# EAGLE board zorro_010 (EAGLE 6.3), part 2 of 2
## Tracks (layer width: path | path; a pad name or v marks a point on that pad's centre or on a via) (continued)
N$8 (continued)
  Top 0.254: 32.56,16.52 33.57,16.52 33.83,16.27 33.83,15.63 33.45,15.25 | 33.45,15.25 33.83,14.87 33.83,14.23 33.57,13.98 32.56,13.98 | 33.45,15.25 33.06,15.25
N$9
  Top 0.152: R7.2 79.3,95.17 79.9,95.77 84.41,95.77 X303.B60
N$10
  Top 0.152: LED1.A R32.2
N$11
  Top 0.152: LED2.A R33.2
N$12
  Top 0.152: LED3.A R34.2
N$13
  Top 0.152: LED4.A R35.2
N$14
  Top 0.152: LED5.A R36.2
N$15
  Top 0.152: LED6.A R37.2
N$18  (via drill 0.25 pad 0.67)
  Top 0.152: R2.2 v78.1,28.17
  Bottom 0.152: v78.1,28.17 79.2,29.27 84.33,29.27 X300.A60
N$19
  Top 0.61: R300.2 26.66,63.94 VR300.5
N$20
  Top 0.152: 3.01,31.11 3.01,29.07 5.55,29.07 5.55,31.11 | 5.55,31.11 3.01,31.11 | 3.01,33.14 3.01,31.11 | 5.55,33.14 3.01,33.14 | 5.55,33.14 5.55,31.11 | 3.01,35.17 3.01,33.14 | 5.55,35.17 3.01,35.17 | 5.55,35.17 5.55,33.14 | 3.01,35.17 3.01,37.2 5.55,37.2 5.55,35.17
N$21  (via drill 0.25 pad 0.67)
  Top 0.152: R3.2 v79.8,53.57
  Bottom 0.152: X301.A60 84.37,52.27 81.1,52.27 v79.8,53.57
N$22  (via drill 0.25 pad 0.67)
  Top 0.152: R9.2 v79.8,56.07
  Bottom 0.152: X301.B60 84.34,57.37 81.1,57.37 v79.8,56.07
N$23
  POWER 0.152: 3.01,37.2 3.01,29.07 5.55,29.07 5.55,37.2 3.01,37.2
N$24
  Bottom 0.254: 35.35,16.52 34.34,16.52 34.08,16.27 34.08,15.63 34.46,15.25 | 34.46,15.25 34.08,14.87 34.08,14.23 34.34,13.98 35.35,13.98 | 34.46,15.25 34.84,15.25
N$31
  GND 0.152: 3.01,37.2 3.01,29.07 5.55,29.07 5.55,37.2 3.01,37.2
N$32A
  Bottom 0.152: 3.01,31.11 3.01,29.07 5.55,29.07 | 3.01,33.14 3.01,31.11 | 3.01,35.17 3.01,33.14 | 3.01,35.17 3.01,37.2 5.55,37.2 5.55,35.17 | 5.55,35.17 5.55,33.14 | 5.55,33.14 5.55,31.11 3.01,31.11 | 5.55,33.14 3.01,33.14 | 5.55,35.17 3.01,35.17
N$40  (via drill 0.25 pad 0.67)
  Top 0.152: R8.2 v76.8,28.17
  Bottom 0.152: X300.B60 84.35,34.37 83,34.37 v76.8,28.17
OPT0
  Top 0.152: R38.2 33.1,59.27 33.1,60.97 35.8,63.67 36.7,63.67 38,62.37 SV3.5 40.9,62.37 44.65,66.12 IC201H.10
OPT1
  Top 0.152: 34.9,59.27 36.2,60.57 SV3.3 39.8,60.57 43.35,64.12 IC201H.14 | 34.9,59.27 | R39.2 34.9,59.27
OPT2
  Top 0.152: R40.2 SV3.1 38.71,58.78 42.55,62.62 IC201H.17
P-AD0
  Top 0.152: IC200L.111 64.05,43.32 64.6,43.87 71,43.87 79.4,52.27 86.91,52.27 X301.A58
  Bottom 0.152: X303.A58 88.16,90.83 88.29,90.7 88.29,88.66 88.1,88.47 88.1,78.51 89.24,77.37 89.24,75.72 88.35,74.83 88.35,72.73 88.16,72.54 X302.A58 88.16,68.29 87.85,67.97 87.85,58.25 89.24,56.86 89.24,55.27 88.35,54.38 88.35,52.22 88.16,52.03 X301.A58 88.16,49.94 88.35,49.74 88.35,37.49 89.24,36.6 89.24,34.82 88.16,33.74 X300.A58
P-AD1
  Top 0.152: IC200L.77 70.35,24.92 74.6,29.17 74.6,30.67 80.8,36.87 86.94,36.87 X300.B58
  Bottom 0.152: X303.B58 88.16,93.81 86.89,92.54 86.89,91.27 87.97,90.19 87.97,88.85 87.7,88.57 87.7,77.96 88.16,77.49 X302.B58 88.16,75.53 87.97,75.33 87.97,73.18 86.89,72.1 86.89,70.83 85.81,69.75 85.81,68.1 86.7,67.21 86.7,57.55 X301.B58 88.16,55.08 87.97,54.89 87.97,52.79 86.89,51.71 86.89,50.38 85.62,49.11 85.62,38.19 X300.B58
P-AD2
  Top 0.152: IC200L.110 64.55,43.22 64.8,43.47 71.2,43.47 77.5,49.77 88.13,49.77 X301.A57
  Bottom 0.152: X300.A57 89.43,31.2 90.7,32.47 90.7,33.74 89.62,34.82 89.62,37.05 89.43,37.23 X301.A57 89.43,49.49 89.24,49.68 89.24,51.71 90.51,52.98 90.51,54.38 89.62,55.27 89.62,57.43 88.67,58.38 88.67,68.16 X302.A57 89.43,69.94 89.24,70.13 89.24,72.16 90.51,73.43 90.51,74.76 89.56,75.72 89.56,77.91 88.5,78.97 88.5,88.37 89.43,89.31 X303.A57
P-AD3
  Top 0.152: IC200L.76 70.45,24.42 75,28.97 75,30.47 78.9,34.37 89.43,34.37 X300.B56
  Bottom 0.152: X303.B56 90.7,93.88 89.43,92.61 89.43,91.27 90.51,90.19 90.51,88.79 90.5,88.77 | X300.B56 90.7,36.79 90.51,36.98 90.51,49.3 89.62,50.19 89.62,51.52 90.89,52.79 90.89,54.89 90.7,55.08 X301.B56 90.7,57.37 90.26,57.81 90.26,67.91 90.51,68.16 90.51,69.75 89.56,70.7 89.56,71.97 90.89,73.3 90.89,75.27 90.7,75.46 X302.B56 90.7,77.94 88.9,79.74 88.9,87.77 89.3,88.17 89.9,88.17 90.5,88.77 | 90.5,88.77 90.5,88.8
P-AD4
  Top 0.152: X301.A55 90.77,47.27 75.6,47.27 68.25,39.92 IC200L.107
  Bottom 0.152: X300.A55 91.97,31.2 93.05,32.28 93.05,33.93 92.16,34.82 92.16,37.62 91.97,37.81 X301.A55 91.97,49.55 92.16,49.74 92.16,51.84 93.05,52.73 93.05,54.38 92.16,55.27 92.16,56.98 92.86,57.68 92.86,67.53 91.97,68.41 X302.A55 91.97,69.94 92.16,70.13 92.16,72.35 93.05,73.24 93.05,74.76 92.16,75.65 92.16,77.64 91.55,78.25 91.55,88.94 X303.A55
P-AD5
  Top 0.152: IC200L.75 70.55,23.92 75.4,28.77 75.4,30.27 77,31.87 90.74,31.87 X300.B55
  Bottom 0.152: X303.B55 91.97,91.27 90.89,90.19 90.89,88.65 90.25,88.01 90.25,78.96 91.78,77.43 91.78,75.27 91.97,75.08 X302.B55 91.97,72.92 91.78,72.73 91.78,70.64 90.89,69.75 90.89,68.16 91.53,67.53 91.53,57.11 91.78,56.86 91.78,54.76 91.97,54.57 X301.B55 91.97,52.54 91.78,52.35 91.78,50.19 90.89,49.3 90.89,37.87 91.78,36.98 91.78,34.31 91.97,34.12 X300.B55
P-AD6
  Top 0.152: X301.A54 93.24,48.02 92.1,46.87 75.8,46.87 68.35,39.42 IC200L.106
  Bottom 0.152: X303.A54 93.24,90.89 93.05,90.7 93.05,88.43 92.9,88.27 92.9,78.54 94.32,77.11 94.32,75.72 93.43,74.83 93.43,73.11 93.24,72.92 X302.A54 93.24,68.41 94.26,67.4 94.26,57.24 94.32,57.17 94.32,55.27 93.43,54.38 93.43,52.22 93.24,52.03 X301.A54 93.24,50 93.05,49.81 93.05,37.63 94.32,36.36 94.32,34.82 93.43,33.93 93.43,31.77 93.24,31.58 X300.A54
P-AD7
  Top 0.152: IC200L.74 70.65,23.42 76.5,29.27 91.5,29.27 92,29.77 92,31.27 93.83,33.11 X300.B53
  Bottom 0.152: X303.B53 94.51,93.43 94.32,93.24 94.32,91.08 93.37,90.13 93.37,88.67 94.25,87.79 94.25,77.82 94.7,77.37 94.7,75.4 94.51,75.21 X302.B53 94.51,72.86 94.32,72.67 94.32,70.76 95.72,69.37 95.72,68.22 95.53,68.03 95.53,57.62 94.7,56.79 94.7,54.76 94.51,54.57 X301.B53 94.51,52.54 94.32,52.35 94.32,50.19 93.43,49.3 93.43,47.72 94.7,46.45 94.7,34.31 94.51,34.12 X300.B53
P-AD8
  Top 0.152: X300.B52 94.16,37.27 80.6,37.27 74.2,30.87 74.2,29.37 70.25,25.42 IC200L.78
  Bottom 0.152: X303.B52 95.78,93.81 94.7,92.73 94.7,91.08 95.91,89.88 95.91,88.48 95.55,88.12 95.55,76.78 X302.B52 95.78,75.59 95.59,75.4 95.59,73.49 94.7,72.61 94.7,70.89 96.8,68.8 96.8,58.19 95.78,57.17 X301.B52 95.78,55.08 95.59,54.89 95.59,52.73 94.7,51.84 94.7,50.19 95.78,49.11 X300.B52
P-AD9
  Top 0.152: X301.A49 97.59,46.47 76,46.47 68.45,38.92 IC200L.105
  Bottom 0.152: X303.A49 99.59,75.97 100.67,74.89 100.67,73.56 99.34,72.22 99.34,70.19 99.59,69.94 X302.A49 99.59,55.46 100.67,54.38 100.67,53.05 99.28,51.65 99.28,49.81 99.59,49.49 X301.A49 99.59,35.01 100.86,33.74 100.86,32.47 99.59,31.2 X300.A49
P-AD10
  Top 0.152: IC200L.79 70.15,25.92 73.8,29.57 73.8,31.07 80.4,37.67 98.84,37.67 X300.B48
  Bottom 0.152: X303.B48 100.86,93.81 99.66,92.61 99.66,91.21 100.67,90.19 100.67,77.75 100.86,77.56 X302.B48 100.86,75.46 101.05,75.27 101.05,73.37 99.72,72.03 99.72,70.7 100.67,69.75 100.67,57.3 100.86,57.11 X301.B48 100.86,55.08 101.05,54.89 101.05,52.86 99.72,51.52 99.72,50.25 100.67,49.3 100.67,35.84 X300.B48
P-AD11
  Top 0.152: X301.A47 99.73,46.07 76.2,46.07 68.55,38.42 IC200L.104
  Bottom 0.152: X303.A47 102.13,88.29 102.32,88.1 102.32,75.78 103.21,74.89 103.21,73.18 102.32,72.29 102.32,70.25 102.13,70.06 X302.A47 102.13,67.91 102.32,67.72 102.32,55.27 103.21,54.38 103.21,53.11 102.32,52.22 102.32,49.68 102.13,49.49 X301.A47 102.13,38.25 102.32,38.06 102.32,34.76 103.21,33.87 103.21,32.22 102.13,31.14 X300.A47
P-AD12
  Top 0.152: X300.B47 102.13,36.34 100.4,38.07 80.2,38.07 73.4,31.27 73.4,29.77 70.05,26.42 IC200L.80
  Bottom 0.152: X303.B47 102.13,91.27 101.05,90.19 101.05,88.48 101.56,87.97 101.56,77.69 101.94,77.3 101.94,75.27 102.13,75.08 X302.B47 102.13,72.8 101.94,72.61 101.94,70.64 101.05,69.75 101.05,67.97 101.44,67.59 101.44,57.3 101.94,56.79 101.94,54.76 102.13,54.57 X301.B47 102.13,52.54 101.94,52.35 101.94,50.19 101.05,49.3 101.05,37.11 101.94,36.22 101.94,34.31 102.13,34.12 X300.B47
P-AD13
  Top 0.152: X301.A46 103.4,47.78 101.3,45.67 76.4,45.67 68.65,37.92 IC200L.103
  Bottom 0.152: X303.A46 103.4,90.89 103.21,90.7 103.21,88.16 103.53,87.84 103.53,78 104.48,77.05 104.48,75.78 103.59,74.89 103.59,72.67 103.4,72.48 X302.A46 103.4,70.44 103.21,70.25 103.21,57.94 104.48,56.67 104.48,55.27 103.59,54.38 103.59,52.67 103.4,52.48 X301.A46 103.4,50.06 103.21,49.87 103.21,37.77 104.48,36.5 104.48,34.76 103.59,33.87 103.59,31.84 103.4,31.65 X300.A46
P-AD14
  Top 0.152: X300.B45 104.67,36.2 102.4,38.47 80,38.47 73,31.47 73,29.97 69.95,26.92 IC200L.81
  Bottom 0.152: X303.B45 104.67,93.43 104.48,93.24 104.48,91.08 103.59,90.19 103.59,88.48 104.86,87.21 104.86,75.14 104.67,74.95 X302.B45 104.67,72.92 104.48,72.73 104.48,70.57 103.59,69.68 103.59,68.22 104.86,66.95 104.86,54.82 104.67,54.63 X301.B45 104.67,52.48 104.48,52.28 104.48,50.13 103.59,49.24 103.59,47.84 104.86,46.57 104.86,34.31 104.67,34.12 X300.B45
P-AD15
  Top 0.152: X301.A44 105.94,47.62 103.6,45.27 76.6,45.27 68.75,37.42 IC200L.102
  Bottom 0.152: X303.A44 105.94,90.89 106.13,90.7 106.13,88.54 106.64,88.03 106.64,77.49 107.02,77.11 107.02,75.65 106.13,74.76 106.13,72.67 105.94,72.48 X302.A44 105.94,70.38 106.13,70.19 106.13,67.97 106.58,67.53 106.58,57.24 107.02,56.79 107.02,55.27 106.13,54.38 106.13,52.48 105.94,52.28 X301.A44 105.94,50 106.13,49.81 106.13,37.11 107.02,36.22 107.02,35.2 105.75,33.93 105.75,30.76 X300.A44
P-AD16
  Top 0.152: X300.A26 127.6,31.77 122.39,31.77 X300.A32 | X301.A32 119.94,49.77 119.2,49.77 118.7,49.27 118.7,47.47 116.1,44.87 76.8,44.87 68.85,36.92 IC200L.101
  Bottom 0.152: X303.A32 121.18,90.83 121.37,90.64 121.37,78.38 120.1,77.11 120.1,75.78 120.99,74.89 120.99,72.61 121.18,72.41 X302.A32 121.18,70.44 121.37,70.25 121.37,68.1 120.74,67.46 120.74,57.43 120.1,56.79 120.1,55.27 120.99,54.38 120.99,52.16 121.18,51.97 X301.A32 121.18,50 121.37,49.81 121.37,47.33 120.1,46.06 120.1,34.82 120.99,33.93 120.99,31.71 121.18,31.52 X300.A32
P-AD17  (via drill 0.3 pad 0.6, 0.3 pad 0.61)
  Top 0.152: X301.A26 128.17,51.01 126.26,52.92 126.26,54.19 125.63,54.82 123.72,54.82 | 123.72,54.82 122.45,54.82 X301.B32 | v123.15,78.51 X302.B32 121.18,73.3 122.26,72.22 122.26,70.64 121.25,69.62 121.25,67.62 v121.69,67.18 | v121.18,45.49 121.18,49.11 122.45,50.38 122.45,51.65 123.72,52.92 123.72,54.82 | X300.B32 117.96,38.87 79.8,38.87 72.6,31.67 72.6,30.17 69.85,27.42 IC200L.82
  Bottom 0.152: X303.B32 121.18,93.81 122.26,92.73 122.26,91.21 123.53,89.94 123.53,88.61 123.15,88.22 v123.15,78.51 | v121.69,67.18 121.82,67.05 121.82,57.68 121.18,57.05 X301.B32 | X300.B32 v121.18,45.49
P-AD18
  Top 0.152: X301.A31 122.45,45.33 121.6,44.47 77,44.47 68.95,36.42 IC200L.100
  Bottom 0.152: X303.A31 122.45,75.97 121.37,74.89 121.37,73.11 122.26,72.22 122.26,70.06 122.45,69.87 X302.A31 122.45,55.46 121.37,54.38 121.37,52.41 122.26,51.52 122.26,49.62 122.45,49.43 X301.A31 122.45,35.01 121.37,33.93 121.37,32.28 122.45,31.2 X300.A31
P-AD19
  Top 0.152: X302.A26 128.17,71.46 126.26,73.37 126.26,74.57 124.3,76.54 X302.B30 | X300.B30 120.1,39.27 79.6,39.27 72.2,31.87 72.2,30.37 69.75,27.92 IC200L.83
  Bottom 0.152: X303.B30 123.72,93.88 122.58,92.73 122.58,91.4 123.85,90.13 123.85,77.75 123.72,77.62 X302.B30 123.72,75.59 123.53,75.4 123.53,73.24 122.64,72.35 122.64,70.57 123.72,69.49 X301.B30 123.72,55.08 123.53,54.89 123.53,52.73 122.64,51.84 122.64,50.19 123.72,49.11 X300.B30
P-AD20
  Top 0.152: X303.A26 128.17,91.91 125.63,89.37 X303.A29 | X301.A29 124.99,46.97 122.1,44.07 77.2,44.07 68.55,35.42 IC200L.98
  Bottom 0.152: X303.A29 124.99,77.37 124.8,77.18 124.8,75.72 123.91,74.83 123.91,73.24 124.8,72.35 124.8,70.06 124.99,69.87 X302.A29 124.99,67.97 124.8,67.78 124.8,55.27 123.91,54.38 123.91,52.79 124.8,51.9 124.8,49.68 124.99,49.49 X301.A29 | X301.A29 124.99,48.41 | X300.A29 124.99,31.2 123.72,32.47 123.72,33.74 124.8,34.82 124.8,48.28 X301.A29
P-AD21
  Top 0.152: X300.B29 124.99,36.28 121.6,39.67 79.4,39.67 68.65,28.92 IC200L.85
  Bottom 0.152: X303.B29 124.99,91.27 126.07,90.19 126.07,78 125.18,77.11 125.18,75.14 124.99,74.95 X302.B29 124.99,72.99 125.18,72.8 125.18,70.64 126.07,69.75 126.07,57.87 125.18,56.98 125.18,54.76 124.99,54.57 X301.B29 124.99,52.54 125.18,52.35 125.18,50.19 126.07,49.3 126.07,47.84 125.18,46.95 125.18,34.31 124.99,34.12 X300.B29
P-AD22
  Top 0.152: X301.A28 126.26,47.14 122.8,43.67 77.4,43.67 68.65,34.92 IC200L.97
  Bottom 0.152: X303.A28 126.26,90.83 126.39,90.7 126.39,88.61 127.09,87.91 127.09,77.75 127.34,77.49 127.34,75.72 126.26,74.64 X302.A28 126.26,70.38 126.39,70.25 126.39,68.1 127.03,67.46 127.03,57.11 127.34,56.79 127.34,55.27 126.26,54.19 X301.A28 126.26,50 126.39,49.87 126.39,37.43 127.34,36.47 127.34,34.82 126.26,33.74 X300.A28
P-AD23
  Top 0.152: X300.B27 127.53,36.34 123.8,40.07 79.2,40.07 68.55,29.42 IC200L.86
  Bottom 0.152: X303.B27 127.53,93.43 127.34,93.24 127.34,91.21 128.61,89.94 128.61,88.48 128.17,88.03 128.17,78 127.72,77.56 127.72,75.21 127.53,75.02 X302.B27 127.53,72.99 127.34,72.8 127.34,70.64 128.61,69.37 128.61,68.03 128.04,67.46 128.04,57.11 127.72,56.79 127.72,54.76 127.53,54.57 X301.B27 127.53,52.54 127.34,52.35 127.34,50.32 128.61,49.05 128.61,47.78 127.72,46.89 127.72,34.31 127.53,34.12 X300.B27
P-AD24
  Top 0.152: X301.A25 124.87,43.27 77.6,43.27 68.75,34.42 IC200L.96
  Bottom 0.152: X303.A25 130.07,75.91 128.99,74.83 128.99,73.18 129.88,72.29 129.88,70.13 130.07,69.94 X302.A25 130.07,55.46 128.99,54.38 128.99,52.67 129.88,51.78 129.88,49.62 130.07,49.43 X301.A25 | X301.A25 130.07,48.22 | X300.A25 130.07,31.2 128.74,32.54 128.74,33.68 130.07,35.01 X301.A25
P-AD25
  Top 0.152: X300.B24 126.52,40.47 79,40.47 68.45,29.92 IC200L.87
  Bottom 0.152: X303.B24 131.34,93.81 130.07,92.54 130.07,91.27 131.15,90.19 131.15,77.69 131.34,77.49 X302.B24 131.34,73.37 130.2,72.22 130.2,70.7 131.15,69.75 131.15,57.24 131.34,57.05 X301.B24 131.34,52.86 130.26,51.78 130.26,50.19 131.15,49.3 131.15,35.84 X300.B24
P-AD26
  Top 0.152: X301.A23 127.01,42.87 77.8,42.87 68.85,33.92 IC200L.95
  Bottom 0.152: X303.A23 132.61,88.35 132.74,88.22 132.74,75.84 133.69,74.89 133.69,73.24 132.8,72.35 132.8,70.19 132.61,70 X302.A23 132.61,67.91 132.8,67.72 132.8,55.27 133.69,54.38 133.69,52.73 132.8,51.84 132.8,49.68 132.61,49.49 X301.A23 132.8,48.28 132.8,34.82 133.69,33.93 133.69,32.28 132.61,31.2 X300.A23
P-AD27
  Top 0.152: X300.B23 132.61,36.26 128,40.87 78.8,40.87 68.35,30.42 IC200L.88
  Bottom 0.152: X303.B23 132.61,91.27 131.53,90.19 131.53,88.61 131.92,88.22 131.92,77.69 132.42,77.18 132.42,75.27 132.61,75.08 X302.B23 132.61,72.99 132.42,72.8 132.42,70.64 131.53,69.75 131.53,68.03 131.98,67.59 131.98,57.17 132.42,56.73 132.42,54.76 132.61,54.57 X301.B23 132.61,52.54 132.42,52.35 132.42,50.19 131.53,49.3 131.53,47.78 132.42,46.89 132.42,34.25 132.61,34.06 X300.B23
P-AD28
  Top 0.152: X301.A22 133.88,47.86 128.5,42.47 78,42.47 68.95,33.42 IC200L.94
  Bottom 0.152: X303.A22 133.88,90.89 133.69,90.7 133.69,78.32 134.96,77.05 134.96,75.78 134.07,74.89 134.07,72.67 133.88,72.48 X302.A22 133.88,70.44 133.69,70.25 133.69,57.87 134.96,56.6 134.96,55.27 134.07,54.38 134.07,52.22 133.88,52.03 X301.A22 133.88,48.09 134.96,47.01 134.96,34.82 134.07,33.93 134.07,31.77 133.88,31.58 X300.A22
P-AD29
  Top 0.152: X300.B21 135.15,36.42 130.3,41.27 78.6,41.27 69.25,31.92 IC200L.91
  Bottom 0.152: X303.B21 135.15,93.43 134.96,93.24 134.96,91.15 134.01,90.19 134.01,88.54 135.03,87.53 135.03,77.49 135.28,77.24 135.28,75.14 135.15,75.02 X302.B21 135.15,72.8 135.03,72.67 135.03,70.7 134.01,69.68 134.01,68.29 134.77,67.53 134.77,57.37 135.34,56.79 135.34,54.76 135.15,54.57 X301.B21 135.15,52.54 134.96,52.35 134.96,50.32 136.23,49.05 136.23,47.78 135.34,46.89 135.34,34.31 135.15,34.12 X300.B21
P-AD30
  Top 0.152: X301.A20 136.42,47.6 130.9,42.07 78.2,42.07 69.05,32.92 IC200L.93
  Bottom 0.152: X303.A20 136.42,90.83 136.55,90.7 136.55,88.16 137.19,87.53 137.19,77.43 137.5,77.11 137.5,75.78 136.61,74.89 136.61,72.67 136.42,72.48 X302.A20 136.42,70.44 136.61,70.25 136.61,66.96 137.5,66.07 137.5,55.33 136.61,54.44 136.61,52.22 136.42,52.03 X301.A20 137,51.01 138.76,49.25 138.76,47.79 137.69,46.72 137.69,34.89 136.42,33.62 X300.A20
P-AD31
  Top 0.152: X300.B20 136.42,36.55 131.3,41.67 78.4,41.67 69.15,32.42 IC200L.92
  Bottom 0.152: X303.B20 136.42,93.81 135.34,92.73 135.34,91.08 136.23,90.19 136.23,77.75 136.42,77.56 X302.B20 136.42,75.53 136.23,75.33 136.23,73.18 135.34,72.29 135.34,70.64 136.23,69.75 136.23,57.3 136.42,57.11 X301.B20 136.42,55.08 136.23,54.89 136.23,52.73 135.34,51.84 135.34,50.44 136.61,49.17 136.61,47.39 136.42,47.2 X300.B20
P-CBE0#
  Top 0.152: X302.A52 94.57,72.67 82.2,72.67 78,68.47 70.7,68.47 69.05,70.12 IC201H.107
  Bottom 0.152: X303.A52 95.78,90.83 96.81,89.8 96.81,77.16 96.86,77.11 96.86,75.72 95.97,74.83 95.97,73.37 95.78,73.18 X302.A52 95.78,70.38 98.13,68.03 98.13,56.67 95.97,54.51 95.97,52.22 95.78,52.03 X301.A52 95.78,50 96.16,49.62 96.16,49.63 96.67,49.12 96.67,36.54 96.99,36.22 96.99,34.89 95.78,33.68 X300.A52
P-CBE1#
  Top 0.152: IC201H.74 70.95,53.62 72.2,54.87 104.72,54.87 X301.B44
  Bottom 0.152: X303.B44 105.94,93.75 104.86,92.67 104.86,91.08 105.75,90.19 105.75,77.81 105.94,77.62 X302.B44 105.94,75.46 105.75,75.27 105.75,73.18 104.86,72.29 104.86,70.57 105.75,69.68 105.75,57.24 105.94,57.05 X301.B44 105.94,55.14 105.75,54.95 105.75,52.98 104.86,52.09 104.86,50.13 105.75,49.24 105.75,35.84 X300.B44
P-CBE2#
  Top 0.152: X301.B33 119.91,57.26 117.9,59.27 73,59.27 70.35,56.62 IC201H.80
  Bottom 0.152: X303.B33 119.91,91.27 120.99,90.19 120.99,88.61 119.72,87.34 119.72,75.14 119.91,74.95 X302.B33 119.91,70.83 120.99,69.75 120.99,68.22 120.04,67.27 120.04,57.37 119.72,57.05 119.72,54.76 119.91,54.57 X301.B33 119.91,50.38 120.99,49.3 120.99,47.97 119.72,46.7 119.72,34.25 119.91,34.06 X300.B33
P-CBE3#
  Top 0.152: X301.B26 125.22,59.67 72.8,59.67 70.25,57.12 IC201H.81
  Bottom 0.152: X303.B26 128.8,93.81 127.72,92.73 127.72,91.34 128.99,90.07 128.99,77.75 128.8,77.56 X302.B26 128.8,75.59 128.61,75.4 128.61,73.18 127.72,72.29 127.72,70.76 128.99,69.49 128.99,57.37 128.8,57.17 X301.B26 128.8,55.08 128.61,54.89 128.61,52.67 127.72,51.78 127.72,50.44 128.99,49.17 128.99,47.2 128.8,47.01 X300.B26
P-CLK0
  Top 0.152: X300.B16 141.5,39.98 141.5,40.67 141.8,40.97 142.5,40.97 142.8,40.67 142.8,38.37 143,38.17 143.9,38.17 144.1,38.37 144.1,48.97 142.8,50.27 142.8,51.57 141.5,52.87 141.5,54.17 140.2,55.47 140.2,56.77 140.9,57.47 140.9,58.27 137.5,61.67 69.5,61.67 67.95,60.12 IC201H.87
P-CLK1
  Top 0.152: IC201H.88 67.85,60.62 69.3,62.07 138.3,62.07 138.9,61.47 146.7,61.47 146.9,61.27 146.9,60.77 146.7,60.57 140.3,60.57 140.1,60.37 140.1,59.97 140.3,59.77 148.6,59.77 148.8,59.57 148.8,59.17 148.6,58.97 141.81,58.97 141.5,58.67 X301.B16
P-CLK2
  Top 0.152: IC201H.101 68.45,67.12 69.5,66.07 131.9,66.07 133.8,67.97 133.8,69.57 134.4,70.17 137.2,70.17 137.6,70.57 137.6,72.37 137.9,72.67 142.3,72.67 142.8,72.17 142.8,70.67 143.5,69.97 144.6,69.97 145.3,70.67 145.3,72.07 146,72.77 147.2,72.77 147.8,72.17 147.8,70.87 148.7,69.97 149.6,69.97 150.4,70.77 150.4,71.97 149.1,73.27 149.1,74.87 148.7,75.27 142.77,75.27 X302.B16
P-CLK3  (via drill 0.25 pad 0.67)
  Top 0.152: v141.1,65.67 139.9,64.47 68.7,64.47 68.55,64.62 IC201H.96
  Bottom 0.152: X303.B16 141.5,93.88 140.3,92.67 140.3,91.17 141.5,89.97 141.5,78.47 140.4,77.37 140.4,75.77 141.5,74.67 141.5,73.27 140.4,72.17 140.4,70.67 141.5,69.57 141.5,66.07 v141.1,65.67
P-DEVSEL#
  Top 0.152: X301.B37 114.83,57.14 113.5,58.47 73.4,58.47 70.55,55.62 IC201H.78 | R13.2 115.7,26.67 115.95,26.92 115.95,28.72 114.83,29.84 X300.B37
  Bottom 0.152: X303.B37 114.83,91.27 115.91,90.19 115.91,88.48 114.64,87.21 114.64,75.14 114.83,74.95 X302.B37 114.83,70.83 115.91,69.75 115.91,68.03 114.64,66.76 114.64,54.7 114.83,54.51 X301.B37 114.83,50.44 115.91,49.36 115.91,47.33 114.64,46.06 114.64,34.19 114.83,34 X300.B37
P-FRAME#
  Top 0.152: X302.A34 118.64,68.02 117.5,66.87 69.9,66.87 68.65,68.12 IC201H.103 | R10.2 119.6,26.57 118.81,27.36 118.81,29.26 118.64,29.43 X300.A34
  Bottom 0.152: X303.A34 118.64,90.83 118.83,90.64 118.83,78.45 117.56,77.18 117.56,75.72 118.64,74.64 X302.A34 118.64,70.44 118.83,70.25 118.83,67.97 119.41,67.4 119.41,58.57 117.56,56.73 117.56,55.27 118.45,54.38 118.45,52.16 118.64,51.97 X301.A34 118.64,50 118.83,49.81 118.83,37.58 117.56,36.31 117.56,34.76 118.64,33.68 X300.A34
P-GNT0#  (via drill 0.25 pad 0.67)
  Top 0.152: v140.2,57.87 136.8,61.27 69.7,61.27 68.05,59.62 IC201H.86 | X300.A17 140.23,26.09 R22.2
  Bottom 0.152: X300.A17 140.23,31.11 141.5,32.37 141.5,33.67 140.2,34.97 140.2,46.37 141.5,47.67 141.5,49.27 140.2,50.57 140.2,51.57 139,52.77 139,54.17 140.2,55.37 v140.2,57.87
P-GNT1#
  Top 0.152: IC201H.83 70.05,58.12 72.4,60.47 132,60.47 135.2,57.27 135.2,55.47 135.8,54.87 138.2,54.87 139,54.07 139,52.77 140.23,51.54 X301.A17 140.23,46.69 R23.2
P-GNT2#
  Top 0.152: IC201H.100 68.35,66.62 69.3,65.67 137.78,65.67 139.28,67.17 R24.2 140.23,67.19 X302.A17
P-GNT3#  (via drill 0.25 pad 0.67)
  Top 0.152: v140,65.57 139.3,64.87 68.9,64.87 68.65,65.12 IC201H.97 | R25.2 140.25,89.35 X303.A17
  Bottom 0.152: X303.A17 140.2,89.33 140.2,77.67 140.05,77.52 140.05,75.72 139.15,74.82 139.15,73.02 140.05,72.12 140.05,70.32 139.15,69.42 139.15,66.72 140,65.87 v140,65.57
P-INTA#  (via drill 0.25 pad 0.67, 0.3 pad 0.61)
  Top 0.152: X300.A6 154.2,33.87 153,35.08 153,36.03 v151.73,37.3 | v152.2,65.57 149.9,63.27 68.7,63.27 68.55,63.12 IC201H.93 | R18.2 151.6,89.94 152.93,91.27 X303.B7
  Bottom 0.152: X303.B7 152.93,91.27 154.01,90.19 154.01,88.73 152.74,87.46 152.74,75.72 151.85,74.83 151.85,73.18 152.74,72.29 152.74,70.13 152.93,69.94 X302.A7 152.93,66.31 v152.2,65.57 151.54,64.91 151.54,61.56 150.58,60.6 150.58,57.17 X301.B8 151.66,55.08 151.47,54.89 151.47,52.73 150.58,51.84 150.58,50.38 151.85,49.11 151.85,37.43 v151.73,37.3
P-INTB#  (via drill 0.3 pad 0.61)
  Top 0.152: v155.47,67.27 155.22,67.53 v152.17,67.53 151.25,67.53 147.4,63.67 68.5,63.67 68.45,63.62 IC201H.94 | R19.2 153,89.3 X303.A7
  Bottom 0.152: X303.A7 152.36,89.37 150.58,87.59 150.58,77.62 X302.B8 151.66,75.53 151.47,75.33 151.47,73.18 150.58,72.29 150.58,70.89 151.85,69.62 151.85,67.84 v152.17,67.53 | v155.47,67.27 155.47,55.46 154.2,54.19 X301.A6 154.2,49.94 154.39,49.74 154.39,37.55 153.12,36.28 153.12,34.25 152.93,34.06 X300.B7
P-INTC#  (via drill 0.25 pad 0.67)
  Top 0.152: v153.8,63.77 152.5,62.47 69.1,62.47 68.75,62.12 IC201H.91 | R20.2 149.65,87.52 149.2,87.97 149.2,89.97 150.4,91.17 150.4,92.47 151.7,93.77 151.7,96.95 X303.B8
  Bottom 0.152: X303.B8 152.3,96.99 154.2,95.08 154.2,93.75 155.47,92.48 155.47,91.21 156.74,89.94 156.74,88.73 155.41,87.4 155.41,75.84 154.2,74.64 X302.A6 154.2,70.51 154.39,70.32 154.39,64.37 v153.8,63.77 153.12,63.1 153.12,54.76 152.93,54.57 X301.B7 152.93,52.54 153.12,52.35 153.12,50.19 154.01,49.3 154.01,37.81 152.74,36.54 152.74,34.82 151.66,33.74 151.66,32.47 152.93,31.2 X300.A7
P-INTD#  (via drill 0.25 pad 0.67)
  Top 0.152: v153.3,64.77 151.4,62.87 68.9,62.87 68.65,62.62 IC201H.92 | X303.A6 154.2,88.47 154.4,88.27 R21.2
  Bottom 0.152: X303.A6 154.2,90.83 154.39,90.64 154.39,88.61 153.12,87.34 153.12,75.21 152.93,75.02 X302.B7 152.93,72.99 153.12,72.8 153.12,70.64 154.01,69.75 154.01,65.49 v153.3,64.77 152.74,64.22 152.74,54.95 151.85,54.06 151.85,52.73 152.74,51.84 152.74,49.68 152.93,49.49 X301.A7 152.93,37.49 151.66,36.22 X300.B8
P-IRDY#
  Top 0.152: X301.B35 117.37,56.9 115.4,58.87 73.2,58.87 70.45,56.12 IC201H.79 | R12.2 118.3,26.77 118.5,26.97 118.5,28.77 117.37,29.9 X300.B35
  Bottom 0.152: X303.B35 117.37,91.27 118.45,90.19 118.45,88.59 117.18,87.32 117.18,75.14 117.37,74.95 X302.B35 117.37,70.83 118.45,69.75 118.45,67.46 118.83,67.08 118.83,58.63 117.18,56.98 117.18,54.7 117.37,54.51 X301.B35 117.37,50.38 118.45,49.3 118.45,47.76 117.18,46.49 117.18,34.31 117.37,34.12 X300.B35
P-LOCK#
  Top 0.152: X301.B39 112.29,54.77 112.45,54.92 112.45,57.72 112.1,58.07 73.6,58.07 70.65,55.12 IC201H.77 | R15.2 112.2,26.37 111.2,27.37 111.2,28.77 112.29,29.87 X300.B39
  Bottom 0.152: X303.B39 112.29,91.27 113.37,90.19 113.37,88.54 112.42,87.59 112.42,87.6 112.1,87.28 112.1,75.14 112.29,74.95 X302.B39 112.29,72.8 112.1,72.61 112.1,70.95 113.37,69.68 113.37,68.1 112.86,67.59 112.86,57.6 112.1,56.84 112.1,54.7 112.29,54.51 X301.B39 112.29,50.38 113.37,49.3 113.37,47.79 112.1,46.52 112.1,34.38 112.29,34.19 X300.B39
P-PAR
  Top 0.152: X302.A43 105.96,70.17 81.6,70.17 79.5,68.07 70.5,68.07 68.95,69.62 IC201H.106
  Bottom 0.152: X303.A43 107.21,88.29 107.4,88.1 107.4,75.65 108.29,74.76 108.29,73.43 107.02,72.16 107.02,70.13 107.21,69.94 X302.A43 107.21,67.97 107.4,67.78 107.4,55.27 108.29,54.38 108.29,53.05 107.02,51.78 107.02,49.62 107.21,49.43 X301.A43 107.34,48.35 107.34,35.01 106.07,33.74 106.07,32.22 107.21,31.07 X300.A43
P-PERR#
  Top 0.152: X301.B40 109.44,57.67 73.8,57.67 70.75,54.62 IC201H.76 | R17.2 110.7,27.07 110.85,27.22 110.85,28.82 109.8,29.87 109.8,31.17 111.02,32.4 X300.B40
  Bottom 0.152: X303.B40 111.02,93.81 109.75,92.54 109.75,91.27 110.83,90.19 111.02,89.99 X302.B40 111.02,75.53 111.21,75.33 111.21,73.3 109.94,72.03 109.94,70.64 110.83,69.75 110.83,57.24 111.02,57.05 X301.B40 111.02,55.08 111.21,54.89 111.21,52.86 109.94,51.59 109.94,50.13 110.83,49.24 110.83,35.84 X300.B40
P-REQ0#
  Top 0.152: X300.B18 138.96,49.01 137.8,50.17 137.8,51.37 136.9,52.27 134.5,52.27 133.9,52.87 133.9,54.17 132.6,55.47 132.6,57.27 129.8,60.07 72.6,60.07 70.15,57.62 IC201H.82
P-REQ1#
  Top 0.152: X301.B18 134.19,60.87 69.9,60.87 68.15,59.12 IC201H.85
P-REQ2#
  Top 0.152: X302.B18 137.69,75.27 137,75.27 136.4,74.67 136.4,73.27 135.8,72.67 133.1,72.67 132.6,72.17 132.6,70.57 131.4,69.37 131.4,67.67 130.2,66.47 69.7,66.47 68.55,67.62 IC201H.102
P-REQ3#  (via drill 0.25 pad 0.67)
  Top 0.152: v139,65.77 138.5,65.27 69.1,65.27 68.75,65.62 IC201H.98
  Bottom 0.152: X303.B18 138.96,93.84 137.7,92.57 137.7,91.27 138.9,90.07 138.9,78.47 137.85,77.42 137.85,75.62 138.8,74.67 138.8,73.47 137.6,72.27 137.6,70.77 138.8,69.57 138.8,65.97 v139,65.77
P-RST#
  Top 0.152: X302.A15 142.8,68.89 142.8,66.37 140.5,64.07 68.5,64.07 68.45,64.12 IC201H.95
  Bottom 0.152: X303.A15 142.8,89.34 142.8,75.87 144,74.67 144,73.17 142.77,71.95 X302.A15 142.8,68.89 142.8,55.47 144.1,54.17 144.1,52.87 142.77,51.55 X301.A15 142.77,35.14 144,33.91 144,32.47 142.77,31.25 X300.A15
P-SERR#
  Top 0.152: X301.B42 107.31,57.27 74,57.27 70.85,54.12 IC201H.75 | R16.2 109.2,26.57 108.5,27.27 108.5,28.57 107.2,29.87 107.2,31.17 108.48,32.46 X300.B42
  Bottom 0.152: X303.B42 108.48,93.88 107.21,92.61 107.21,91.21 108.48,89.94 X302.B42 108.48,75.53 108.67,75.33 108.67,73.3 107.4,72.03 107.4,70.57 108.48,69.49 X301.B42 108.48,54.82 108.67,54.63 108.67,52.92 107.4,51.65 107.4,50 108.48,48.92 X300.B42
P-STOP#
  Top 0.152: X302.A38 113.56,68.34 112.9,67.67 70.3,67.67 68.85,69.12 IC201H.105 | R14.2 113.7,26.97 113.56,27.11 X300.A38
  Bottom 0.152: X303.A38 113.56,90.89 113.75,90.7 113.75,78.64 112.48,77.37 112.48,75.72 113.56,74.64 X302.A38 113.56,70.44 113.75,70.25 113.75,57.92 112.48,56.65 112.48,55.27 113.37,54.38 113.37,52.09 113.56,51.9 X301.A38 113.56,50 113.75,49.81 113.75,37.63 113.12,37 113.12,36.98 112.48,36.35 112.48,34.82 113.56,33.74 X300.A38
P-TCK
  Top 0.152: X300.B2 159.28,49.06 160.6,50.37 160.6,51.57 159.28,52.89 X301.B2 159.28,69.56 160.7,70.97 160.7,71.77 159.28,73.19 X302.B2 159.28,76.56 159.98,76.56 164,80.57 164,87.57 | 164,87.57 164,88.27 160.7,91.57 160.7,92.17 159.28,93.59 X303.B2 | R30.2 163.95,87.52 164,87.57
  Bottom 0.152: X300.B2 159.28,32.46 158,31.17 158,30.07 156.8,28.87 156.8,27.27 155.5,25.97 152.1,25.97 151.2,25.07 SV1.4
P-TDI  (via drill 0.25 pad 0.67)
  Top 0.152: X303.A4 156.74,87.72 v156.6,87.57 156.95,87.22 R29.2 | v156,79.67 154.9,79.67 153,77.77 153,76.07 151.7,74.77 151.7,73.37 152.9,72.17 152.9,70.87 153.6,70.17 156.1,70.17 156.7,69.57 156.7,61.27 152.9,57.47 152.9,55.47 151.7,54.27 151.7,52.97 152.9,51.77 152.9,50.37 151.7,49.17 151.7,40.77 v147.9,36.97
  Bottom 0.152: v156.6,87.57 156,86.97 v156,79.67 | v147.9,36.97 147.9,35.17 146.6,33.87 146.6,32.47 147.8,31.27 147.8,29.87 146.6,28.67 146.6,25.67 146.12,25.19 SV1.2
P-TDI1  (via drill 0.25 pad 0.67)
  Top 0.152: X302.A4 156.11,71.46 154.2,73.37 154.2,74.67 155.4,75.87 155.4,77.37 v156.7,78.67
  Bottom 0.152: X303.B4 156.74,93.93 158,92.67 158,91.27 159.3,89.97 159.3,88.97 156.7,86.37 v156.7,78.67
P-TDI2
  Bottom 0.152: X302.B4 156.74,73.42 155.5,72.17 155.5,70.77 156.7,69.57 156.7,58.47 158,57.17 158,55.37 156.8,54.17 156.8,51.07 X301.A4
P-TDI3  (via drill 0.25 pad 0.67)
  Top 0.152: X301.B4 156.12,56.09 154.2,54.17 154.2,52.97 155.4,51.77 155.4,50.47 156.7,49.17 v156.7,39.07
  Bottom 0.152: v156.7,39.07 158,37.77 158,34.97 156.74,33.72 X300.A4
P-TDO
  Bottom 0.152: X300.B4 155.57,34.47 155,34.47 154.2,33.67 154.2,32.47 | 154.2,32.47 154.2,32.27 | 154.2,32.47 155.5,31.17 155.5,29.87 | 155.5,29.87 155.5,29.77 | 155.5,29.87 154.2,28.57 154.2,27.07 153.6,26.47 150.1,26.47 148.66,25.03 SV1.3
P-TMS
  Top 0.152: X300.A3 158.01,31.16 156.7,32.47 156.7,33.67 158,34.97 158,48.46 X301.A3 158.01,51.66 156.8,52.87 156.8,54.17 158,55.37 158,68.91 X302.A3 158.01,72.06 156.7,73.37 156.7,74.57 158,75.87 158,77.47 159.4,78.87 161.7,78.87 163.6,80.77 163.6,86.57 163.3,86.87 161.6,86.87 | X303.A3 158.01,88.46 159.6,86.87 161.6,86.87 | 161.6,86.87 R28.2
  Bottom 0.152: SV1.5 153.74,25.01 154.2,25.47 155.8,25.47 158.01,27.69 X300.A3
P-TRDY#
  Top 0.152: X302.A36 116.1,68.18 115.2,67.27 70.1,67.27 68.75,68.62 IC201H.104 | R11.2 117,26.57 116.3,27.27 116.3,29.17 116.1,29.37 X300.A36
  Bottom 0.152: X303.A36 116.1,90.83 116.23,90.7 116.23,78.57 115.02,77.37 115.02,75.65 116.1,74.57 X302.A36 116.1,70.44 116.29,70.25 116.29,67.33 115.6,66.64 115.6,57.68 115.02,57.11 115.02,55.27 115.91,54.38 115.91,52.22 116.1,52.03 X301.A36 116.1,50 116.29,49.81 116.29,37.74 115.02,36.47 115.02,34.76 116.1,33.68 X300.A36
P-TRST  (via drill 0.25 pad 0.67)
  Top 0.152: X300.A1 160.55,31.12 159.3,32.37 159.3,33.77 v160.9,35.37 | X303.A1 160.4,89.22 R31.2
  Bottom 0.152: v160.9,35.37 160.9,36.67 159.5,38.07 159.5,47.42 X301.A1 159.9,48.48 158,50.37 158,51.57 159.3,52.87 159.3,54.17 160.7,55.57 160.7,68.78 X302.A1 159.85,68.92 158,70.77 158,72.07 159.3,73.37 159.3,74.57 158,75.87 158,86.81 X303.A1 | SV1.6 156.28,25.15 157.5,26.37 158.9,26.37 X300.A1
READ  (via drill 0.25 pad 0.67)
  Top 0.152: CON100.68 87.56,8.01 v86.5,9.07 | v49.9,23.07 49.55,23.42 IC200L.35 44.55,23.42 44.3,23.67 41.2,23.67 36.2,28.67 36.2,29.97 36.2,53.87 42.95,60.62 IC201H.21
  Bottom 0.152: v49.9,23.07 50.6,22.37 50.6,21.17 56.4,15.37 80.2,15.37 v86.5,9.07
SA2  (via drill 0.25 pad 0.67)
  Top 0.152: v138.9,8.37 138.4,8.37 138.2,8.57 136.3,8.57 129.5,15.37 59.3,15.37 56.05,18.62 IC200L.54 56.05,21.62 55.8,21.87 55.8,23.67 56.7,24.57 56.7,31.07 58.7,33.07 58.7,36.27 v58.5,36.47 | IC201H.15 46.55,63.62 46.6,63.67 v47.5,63.67
  Bottom 0.152: CON100.27 138.4,4.09 138.4,7.87 v138.9,8.37 | v58.5,36.47 58.2,36.77 58.2,38.47 58.9,39.17 58.9,48.67 57.8,49.77 57.8,53.87 48,63.67 v47.5,63.67
SA3  (via drill 0.25 pad 0.67)
  Top 0.152: CON100.26 140.9,7.87 139.7,9.07 136.4,9.07 129.7,15.77 60.9,15.77 57.05,19.62 IC200L.56 57.05,21.72 57.1,21.77 57.1,30.87 59.1,32.87 59.1,37.07 v58.9,37.27 | IC201H.13 46.65,64.62 v46.9,64.37
  Bottom 0.152: v58.9,37.27 58.6,37.57 58.6,38.27 59.3,38.97 59.3,48.87 58.2,49.97 58.2,54.07 47.9,64.37 v46.9,64.37
SA4  (via drill 0.25 pad 0.67)
  Top 0.152: CON100.24 143.44,7.93 141.9,9.47 136.6,9.47 129.9,16.17 61.1,16.17 57.55,19.72 IC200L.57 57.55,21.62 57.5,21.67 57.5,30.67 59.5,32.67 59.5,37.87 v59.3,38.07 | IC201H.12 47.45,65.12 v47.5,65.07
  Bottom 0.152: v59.3,38.07 59.7,38.47 59.7,49.07 58.6,50.17 58.6,54.27 47.8,65.07 v47.5,65.07
SA5  (via drill 0.25 pad 0.67)
  Top 0.152: v145,8.27 144.3,8.97 143.8,8.97 142.5,10.27 137,10.27 130.3,16.97 61.5,16.97 58.55,19.92 IC200L.59 58.55,21.72 58.3,21.97 58.3,30.27 60.3,32.27 60.3,36.27 v60.5,36.47 | IC201H.9 47.35,66.62 v47.5,66.47
  Bottom 0.152: CON100.21 146,4.07 146,7.57 145.3,8.27 v145,8.27 | v60.5,36.47 60.8,36.77 60.8,37.57 60.5,37.87 60.5,49.47 59.4,50.57 59.4,54.67 47.6,66.47 v47.5,66.47
SA6  (via drill 0.25 pad 0.67)
  Top 0.152: v144,8.27 143.8,8.27 142.2,9.87 136.8,9.87 130.1,16.57 61.3,16.57 58.05,19.82 IC200L.58 58.05,21.72 57.9,21.87 57.9,30.47 59.9,32.47 59.9,37.07 v60.1,37.27 | IC201H.11 46.75,65.62 v46.9,65.77
  Bottom 0.152: CON100.23 143.4,4.09 143.4,7.67 v144,8.27 | v60.1,37.27 60.1,49.27 59,50.37 59,54.47 47.7,65.77 v46.9,65.77
SA7  (via drill 0.25 pad 0.67)
  Top 0.152: CON100.28 138.36,7.81 138,8.17 136.1,8.17 129.3,14.97 59.1,14.97 55.55,18.52 IC200L.53 55.55,21.62 55.4,21.77 55.4,23.87 56.3,24.77 56.3,31.27 58.3,33.27 58.3,35.47 v58.1,35.67 | IC201H.16 46.75,63.12 v46.9,62.97
  Bottom 0.152: v58.1,35.67 57.8,35.97 57.8,38.67 58.5,39.37 58.5,48.47 57.4,49.57 57.4,53.67 48.1,62.97 v46.9,62.97
SD0  (via drill 0.25 pad 0.67)
  Top 0.152: IC200L.15 46.85,33.42 v47.2,33.77
  Bottom 0.152: v47.2,33.77 47.1,33.67 47.1,24.67 47.6,24.17 47.6,21.17 55.4,13.37 73,13.37 77.4,8.97 77.4,4.07 CON100.75
SD1  (via drill 0.25 pad 0.67)
  Top 0.152: IC200L.13 44.75,34.42 44.2,33.87 v44.2,33.47
  Bottom 0.152: CON100.77 74.9,4.09 74.9,8.97 71.3,12.57 55,12.57 51.6,15.97 50.3,15.97 45.8,20.47 45.8,31.57 44.2,33.17 v44.2,33.47
SD2  (via drill 0.25 pad 0.67)
  Top 0.152: IC200L.11 44.55,35.42 44.2,35.07 43.3,35.07 42.9,34.67 42.9,33.57 v43,33.47
  Bottom 0.152: CON100.79 72.3,4.07 72.3,8.87 69.4,11.77 54.6,11.77 51.2,15.17 49.9,15.17 45,20.07 45,29.87 43,31.87 v43,33.47
SD3  (via drill 0.25 pad 0.67)
  Top 0.152: v69.5,9.37 69.1,9.77 52.8,9.77 v52.6,9.97
  Top 0.305: R100.1 52.1,10.47 v52.6,9.97
  Bottom 0.152: 69.8,4.07 CON100.81 69.78,9.09 v69.5,9.37
SD3X  (via drill 0.25 pad 0.66, 0.25 pad 0.67)
  Top 0.152: IC200L.9 44.45,36.42 43.9,35.87 42.7,35.87 v42.3,35.47 | v48,15.57 48.7,14.87 D100.3 | v50.1,12.47
  Top 0.305: R100.2 v50.1,12.47 D100.3
  Bottom 0.152: v42.3,35.47 41.7,34.87 41.7,31.97 43.1,30.57 43.1,22.97 44.2,21.87 44.2,19.37 v48,15.57
SD4  (via drill 0.25 pad 0.67)
  Top 0.152: IC200L.6 44.65,37.92 44,38.57 v43.3,38.57
  Bottom 0.152: CON100.83 67.2,4.09 67.2,9.07 65.7,10.57 54.2,10.57 50.8,13.97 48,13.97 42.3,19.67 42.3,30.17 40.9,31.57 40.9,35.47 43.1,37.67 43.1,38.37 v43.3,38.57
SD5  (via drill 0.25 pad 0.67)
  Top 0.152: CON100.86 64.7,7.67 v63.4,8.97 | IC200L.4 44.65,38.92 43.6,39.97 v42.3,39.97
  Bottom 0.152: v42.3,39.97 41.7,39.97 40.1,38.37 40.1,31.17 41.5,29.77 41.5,19.27 47.6,13.17 50.6,13.17 54,9.77 62.7,9.77 63.5,8.97 v63.4,8.97
SD6  (via drill 0.25 pad 0.67)
  Top 0.152: CON100.84 67.24,7.73 v66,8.97 | IC200L.5 44.65,38.42 43.8,39.27 v42.8,39.27
  Bottom 0.152: v42.8,39.27 41.6,39.27 40.5,38.17 40.5,31.37 41.9,29.97 41.9,19.47 47.8,13.57 50.7,13.57 54.1,10.17 64.8,10.17 v66,8.97
SD7  (via drill 0.25 pad 0.67)
  Top 0.152: CON100.82 69.78,7.79 68.8,8.77 v68.5,8.77 | v43.8,37.87 44.2,37.87 44.65,37.42 IC200L.7
  Bottom 0.152: v43.8,37.87 43.8,37.77 41.3,35.27 41.3,31.77 42.7,30.37 42.7,22.67 43.8,21.57 43.8,18.77 48.2,14.37 50.9,14.37 54.3,10.97 66.3,10.97 v68.5,8.77
SENSEZ3  (via drill 0.25 pad 0.67)
  Top 0.152: IC200L.3 44.65,39.42 43.4,40.67 v41.8,40.67 41,40.67 40.6,41.07 40.6,42.27 41.95,43.62 R1.1 43.1,52.97 44.25,54.12 IC201H.34
  Bottom 0.152: v41.8,40.67 39.7,38.57 39.7,30.97 41.1,29.57 41.1,18.97 47.4,12.67 48.6,12.67 51.9,9.37 55.5,9.37 57.08,7.79 CON100.91 57.1,4.07
SYSCLK  (via drill 0.25 pad 0.67)
  Top 0.152: R202.2 28.95,23.92 29,23.97 R201.2 29.5,23.97 34,28.47 34,53.57 v36.3,55.87 | IC201H.30 44.05,56.12 v44,56.07
  Bottom 0.152: v44,56.07 36.5,56.07 v36.3,55.87
SYSCLK_OSC
  Top 0.152: R201.1 27.65,24.82 26.3,26.17 26.27,26.2 26.21,26.26 Q202.8 26.21,28.46 Q201.5
SYSCLK_PLL
  Top 0.152: IC220.5 26.41,19.08 26.4,19.07 26.4,20.57 27.65,21.82 R202.1
TCK  (via drill 0.25 pad 0.67)
  Top 0.152: RA202.8 17.3,48.97 18.4,47.87 21.7,47.87 22.9,49.07 22.9,49.97 22.2,50.67 20.4,50.67 CON200.1 | IC200L.67 62.55,22.52 62.4,22.67 62.4,39.57 v62,39.97 48.2,39.97 46,42.17 46,50.37 v45.6,50.77 | IC201H.67 62.55,48.12 v62.4,47.97
  Bottom 0.152: v62.4,47.97 62.3,47.87 62.3,44.07 61.7,43.47 61.7,40.27 v62,39.97 | v45.6,50.77 45.5,50.87 20.59,50.87 CON200.1
TDI  (via drill 0.25 pad 0.67)
  Top 0.152: CON200.9 28.73,49.4 27.4,48.07 23.2,48.07 22.2,47.07 18,47.07 17.7,47.37 RA202.6 | IC200L.63 60.55,22.02 61.6,23.07 61.6,38.17 60.6,39.17 48,39.17 45.2,41.97 45.2,48.77 v44.9,49.07
  Bottom 0.152: CON200.9 44.57,49.4 v44.9,49.07
TDO
  Top 0.152: CON200.3 20.53,48.27 18.7,48.27 17.8,49.17 17.8,52.57 18.4,53.17 24.5,53.17 36.2,64.87 36.2,74.87 39.1,77.77 56.5,77.77 57.4,76.87 57.4,75.07 58.55,73.92 IC201H.122
TDO-TDI
  Top 0.152: IC200L.122 58.55,46.02 58.6,46.07 58.6,47.87 60.55,49.82 IC201H.63
TMS  (via drill 0.25 pad 0.67)
  Top 0.152: CON200.5 23.93,49.4 22,47.47 18.2,47.47 17.5,48.17 RA202.7 | IC200L.65 61.55,22.22 62,22.67 62,38.67 v61.6,39.07 61.1,39.57 48.1,39.57 45.6,42.07 45.6,49.37 v44.9,50.07 | IC201H.65 61.55,49.62 61.1,49.17 v61.1,47.17
  Bottom 0.152: v61.1,47.17 61.9,46.37 61.9,44.27 61.3,43.67 61.3,39.37 v61.6,39.07 | CON200.5 25.27,50.47 44.5,50.47 v44.9,50.07
VCC  (via drill 0.25 pad 0.66, 0.25 pad 0.67)
  Top 0.813: 11.7,21.37 R210.1 | v11.7,20.67 11.7,21.37 | v11.7,22.07 11.7,21.37
  Top 1.27: VR100.3 163.12,18.66 164.5,17.27 C12.1 v164.5,10.87 v165.4,9.97 v166.3,9.07 CON100.5
  Bottom 0.813: 26.74,52.01 26.8,52.07 | 26.74,52.01 CON200.8 26.7,51.97 | 26.7,51.97 26.67,51.94 CON200.6 22.47,53.67 14.9,53.67 11.7,50.47 v11.7,22.07 v11.7,20.67 11.7,14.77 16.8,9.67 45.1,9.67 v46,8.77 | 26.7,51.97 26.74,52.01
  Bottom 1.27: CON100.5 v166.3,9.07 v164.5,10.87
  pour POWER: 173.6,7.57 173.6,6.27 44.7,6.27 44.7,9.17 46.4,9.17 46.4,7.57 165.8,7.57 165.8,9.37 166.8,9.37 166.8,7.57
VDD  (via drill 0.25 pad 0.66, 0.25 pad 0.67)
  Top 0.254: RA202.2 14.3,48.17 14,47.87 v14,47.37 | v14,47.37 RA202.3 | v14,47.37 14,46.87 14.3,46.57 RA202.4
  Top 0.305: v49.17,41.17 49.05,41.3 IC200L.141 C204.2 | v56.17,41.17 56.05,41.3 IC200L.127 C201.2 | v46.92,37.05 46.8,36.92 IC200L.8 43.6,36.92 C202.2 | v65.7,28.55 65.83,28.42 IC200L.84 69.25,28.42 C205.2 | C207.2 68.25,22.62 67.95,22.92 IC200L.73 65.92,22.92 v65.8,23.05 | v49.92,22.17 50.05,22.05 IC200L.42 C208.2 50.05,18.92 | v56.42,22.17 56.55,22.05 IC200L.55 56.55,19.12 56.8,18.87 C209.2 | 65.95,42.42 65.9,42.47 | 65.9,42.47 v65.88,42.47 | IC200L.109 65.85,42.42 65.9,42.47 | IC200L.37 47.5,20.97 v46.52,20.97 46.5,20.97 46.45,20.92 C206.2 | IC200L.1 44.85,40.42 44.5,40.77 v44.5,41.15 44.5,41.17 | v50.2,52.47 50.05,52.32 IC201H.42 50.05,49.52 C9.2 | v56.4,52.47 56.55,52.32 IC201H.55 56.55,49.52 C10.2 | v65.8,53.27 65.95,53.12 IC201H.73 67.95,53.12 68.2,52.87 C5.2 | v47,67.37 46.75,67.12 IC201H.8 43.95,67.12 C2.2 | v46.8,70.47 46.65,70.62 IC201H.1 45.55,71.92 C1.2 | v48.9,71.17 49.05,71.32 IC201H.141 49.05,74.12 C7.2 | v55.9,71.27 56.05,71.42 IC201H.127 56.05,74.12 C8.2 | v64.9,71.27 65.05,71.42 IC201H.109 65.1,72.57 C3.2 | v65.8,58.77 65.95,58.62 IC201H.84 68.75,58.62 C4.2 | IC201H.37 47.55,49.92 v47.6,49.87 | C200.2 44.4,42.17 R1.2
  Top 0.406: C203.2 65.95,42.42 | C200.2 44.35,41.32 44.5,41.17 | 157.3,12.37 R101.2 | C6.2 47.4,49.67 v47.6,49.87 | R37.1 R36.1 R35.1 R34.1 R33.1 R32.1 v43.7,75.57 | R39.1 R40.1 | R39.1 v31.8,56.17 | R38.1 R39.1
  Top 0.813: R209.1 v10,23.47 v9,23.47
  other vias: 145.5,19.37 146.8,19.37 148.1,19.37 149.4,19.37 146.8,18.07 148.1,18.07 149.4,18.07 146.8,14.67 148.1,14.67 149.4,14.67 145.5,13.37 146.8,13.37 148.1,13.37 149.4,13.37 152.8,12.17 154.1,12.17 155.4,12.17 156.7,12.17 150.2,12.17 151.5,12.17
  pour POWER (isolate 0.254): 0.46,54.77 0.5,38.47 0.5,9.27 13.4,9.27 13.4,38.47 29,38.47 29,9.67 46.86,9.67 46.86,8.07 165.3,8.07 165.3,9.77 167.2,9.87 167.2,8.07 172.65,8.07 172.7,8.07 172.7,21.07 75.6,21.07 73.9,21.07 73.9,83.67 0,83.67
  pour Top (no thermals): 157.5,19.07 157.5,12.17 156.9,11.57 149.7,11.57 148.3,12.97 145.4,12.97 144.5,13.87 144.5,18.87 145.4,19.77 156.8,19.77
VPP  (via drill 0.25 pad 0.66, 0.25 pad 0.67)
  Top 0.305: v22.8,10.97 C220.2 C221.2 23.86,12.11 IC220.2 23.86,19.04 23.9,19.07 IC220.7 | R204.2 v22.6,20.77 | R205.2 v22.6,22.97
  Top 0.406: Q201.8 26.21,42.28 Q202.14 26.21,43.06 26.2,43.07 26.23,43.1 26.3,43.1 C231.2 C230.2 25,44.67 21.1,40.77 v21.1,37.67
  Top 0.813: R210.2 15.05,23.42 15.1,23.47 R209.2 15.05,25.12 v15.1,25.17 v14.3,25.97
  pour POWER (isolate 0.254): 14.1,37.97 28.3,37.97 28.3,8.77 14.1,8.77

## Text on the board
Top: 1 | G | I | O | C | M | R | V | 1
GND: 2
POWER: 3
Bottom: 4
Document: 44.6mm | 44.6mm | 44.6mm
